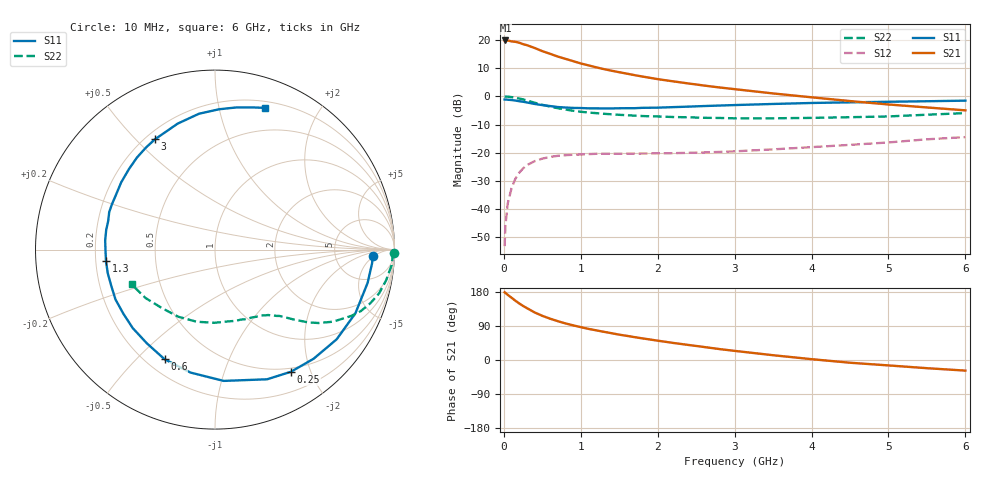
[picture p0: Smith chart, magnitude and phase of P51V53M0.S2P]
! SIEMENS Small Signal Semiconductors
! BFP183
! Si NPN RF Bipolar Junction Transistor in SOT143
! VCE = 1.5 V  IC = 3 mA
! Common Emitter S-Parameters:  March  1996
# GHz  S  MA  R  50
!  f  S11  S21  S12  S22
! GHz  MAG  ANG  MAG  ANG  MAG  ANG  MAG  ANG
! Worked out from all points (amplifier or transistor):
!   36 points, 10 MHz to 6 GHz, reference 50 ohm
!   highest |S21| = 19.8 dB at 20 MHz (marker M1)
!   |S21| within 3 dB of that: start of sweep to 429.7 MHz
!   unconditionally stable (mu >= 1): 1.824 GHz to 5.952 GHz
!   at 250 MHz: K = 0.16, MSG = 22.0 dB, |S12| = -25.6 dB
!   at 1.4 GHz: K = 0.80, MSG = 14.7 dB, |S12| = -20.4 dB
!   at 6 GHz: K = 0.99, MSG = 4.7 dB, |S12| = -14.5 dB
!   S11 on the Smith chart (normalised r, x): 10 MHz: 14, -5; 250 MHz: 0.45, -1.71; 600 MHz: 0.27, -0.61; 1.3 GHz: 0.24, -0.05; 3 GHz: 0.24, +0.57; 6 GHz: 0.26, +1.38
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0.01  0.8801 -2.4  9.697 178.7  0.0022 81.4  0.9965 -1.0
0.02  0.8784 -5.0  9.792 177.4  0.005 84.4  0.9911 -2.1
0.05  0.8703 -12.3  9.789 172.0  0.0125 86.1  0.9874 -5.1
0.15  0.8422 -36.4  9.263 156.5  0.0345 69.6  0.9465 -14.9
0.2  0.8195 -47.9  8.931 149.2  0.0442 65.2  0.9153 -19.1
0.25  0.8015 -58.1  8.42 142.7  0.0526 59.1  0.8814 -22.9
0.3  0.7787 -68.1  8.076 136.9  0.0602 54.7  0.8437 -26.0
0.4  0.7332 -86.2  7.204 125.5  0.0708 46.5  0.7708 -31.4
0.5  0.6986 -101.3  6.33 116.6  0.0785 39.8  0.7078 -35.3
0.6  0.6723 -114.7  5.689 109.1  0.0842 35.1  0.6589 -38.0
0.7  0.6456 -126.0  5.077 102.5  0.088 31.3  0.6166 -40.0
0.8  0.6335 -136.3  4.625 96.6  0.0903 28.4  0.5831 -41.8
0.9  0.6231 -145.0  4.21 91.5  0.0922 25.9  0.5547 -43.3
1.1  0.6122 -160.9  3.542 82.1  0.0945 22.2  0.5155 -45.8
1.3  0.6107 -173.9  3.04 74.4  0.0957 19.6  0.4902 -48.4
1.7  0.6161 164.9  2.375 60.3  0.0964 18.1  0.4538 -53.9
2.2  0.6432 144.3  1.844 45.1  0.0982 18.1  0.4295 -61.9
3  0.6997 118.6  1.34 24.1  0.1057 21.2  0.4076 -78.5
3.5  0.7321 106.5  1.125 12.6  0.1146 22.9  0.4078 -90.4
4.5  0.7823 88.3  0.824 -7.2  0.1377 23.0  0.4263 -118.7
5.5  0.8181 75.6  0.635 -21.6  0.1729 20.6  0.4719 -145.2
6  0.8381 70.4  0.564 -28.0  0.1891 16.9  0.5039 -157.4
